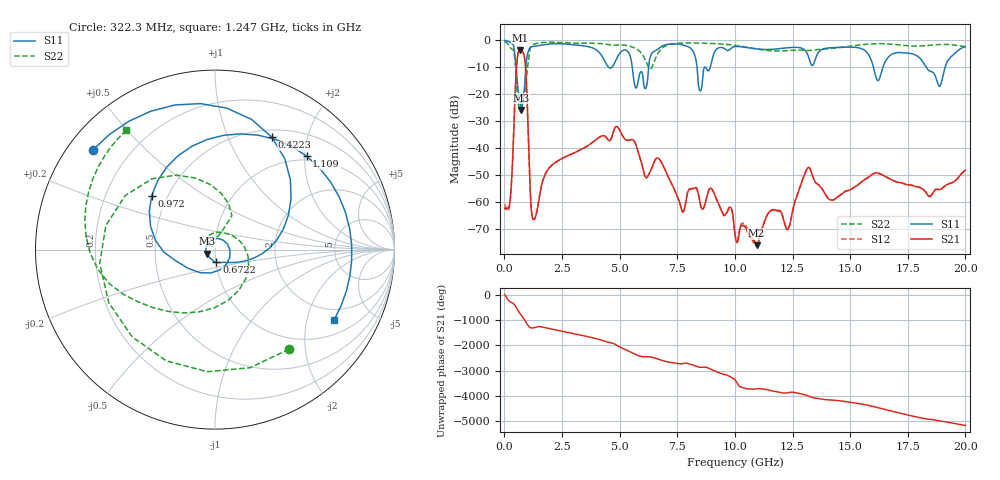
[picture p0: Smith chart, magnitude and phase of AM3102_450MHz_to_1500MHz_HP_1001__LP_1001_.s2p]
!Agilent Technologies,E8364B,MY43040894,A.07.50.67
!Agilent E8364B: A.07.50.67
!Date: Thursday, January 11, 2018 06:03:41
!Correction: S11(Full 2 Port(1,2))
!S21(Full 2 Port(1,2))
!S12(Full 2 Port(1,2))
!S22(Full 2 Port(1,2))
!S2P File: Measurements: S11, S21, S12, S22:
# Hz S  dB  R 50
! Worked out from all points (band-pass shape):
!   1601 points, 10 MHz to 20 GHz, reference 50 ohm
!   highest |S21| = -3.54 dB at 697.2 MHz (marker M1); lowest = -76.2 dB at 10.94 GHz (marker M2)
!   |S21| within 3 dB of the highest: 563.5 MHz to 876.3 MHz (312.9 MHz wide, 43.5 % of centre)
!   lowest |S11| = -25.9 dB at 722.1 MHz (marker M3), VSWR 1.11, Z = 45.6 - j2.05 ohm
!   |S11| at or under -10 dB: 506 MHz to 929.8 MHz (423.8 MHz wide, 59 % of centre); 5.548 GHz to 6.255 GHz (706.9 MHz wide, 12 % of centre); 18.3 GHz to 19.12 GHz (823 MHz wide, 4.4 % of centre)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
!   |S22| runs from -25.3 to -0.5 dB; largest |S21 - S12| = 0.00079
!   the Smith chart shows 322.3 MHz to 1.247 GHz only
!   S11 on the Smith chart (normalised r, x): 322.3 MHz: 0.07, +0.35; 422.3 MHz: 0.59, +1.46; 672.2 MHz: 1.01, -0.14; 972 MHz: 0.41, +0.31; 1.109 GHz: 0.92, +2.04; 1.247 GHz: 1.54, -2.95
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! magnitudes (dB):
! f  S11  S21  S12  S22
! 10 MHz  0.0  -62.3  -60.7  -0.5
! 322.3 MHz  -1.1  -50.8  -50.8  -3.2
! 422.3 MHz  -3.1  -29.2  -29.4  -4.7
! 672.2 MHz  -22.9  -3.6  -3.6  -25.2
! 697.2 MHz  -24.8  -3.5  -3.5  -25.2
! 722.1 MHz  -25.9  -3.6  -3.6  -24.3
! 972 MHz  -6.7  -18.9  -18.9  -12.5
! 1.109 GHz  -2.7  -53.4  -53.2  -3.6
! 1.247 GHz  -2.3  -66.4  -66.6  -1.6
! 3.346 GHz  -2.0  -40.4  -40.5  -1.1
! 4.895 GHz  -6.4  -32.1  -32.1  -1.7
! 6.119 GHz  -17.9  -50.8  -50.7  -7.4
! 6.682 GHz  -3.1  -43.8  -43.8  -4.5
! 7.719 GHz  -1.7  -63.6  -63.5  -1.0
! 8.081 GHz  -3.0  -55.3  -55.2  -1.0
! 8.493 GHz  -18.8  -60.6  -60.8  -1.0
! 10.01 GHz  -2.3  -71.9  -71.7  -1.9
! 10.94 GHz  -3.2  -76.2  -75.9  -3.2
! 13.34 GHz  -9.3  -49.6  -49.5  -3.7
! 16.68 GHz  -6.1  -51.3  -51.2  -1.4
! 18.88 GHz  -17.1  -55.4  -55.4  -1.6
! 20 GHz  -2.4  -48.3  -48.5  -2.3
